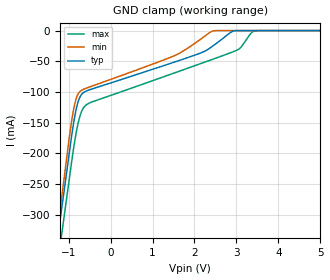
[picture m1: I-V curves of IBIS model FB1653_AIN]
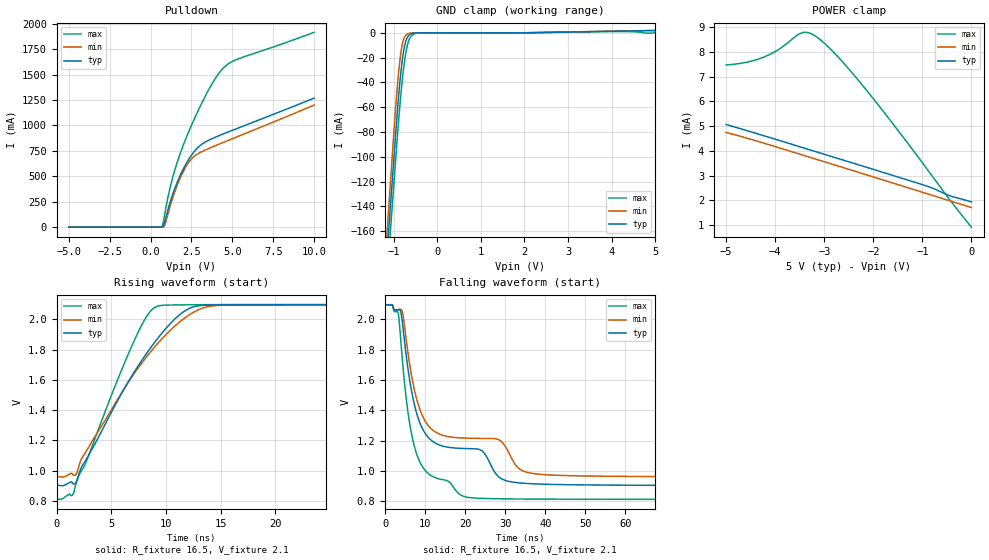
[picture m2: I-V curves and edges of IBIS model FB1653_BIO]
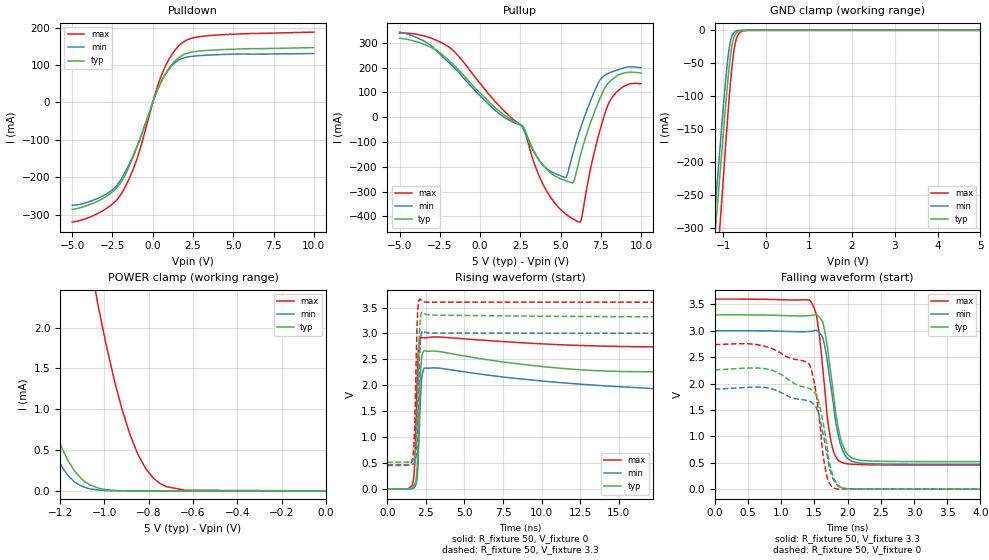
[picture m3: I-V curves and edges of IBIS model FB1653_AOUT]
| TEXAS INSTRUMENTS INCORPORATED
| Standard Linear and Logic Group
| IBIS Model of SN74FB1653
| 17-BIT LVTTL/BTL UNIVERSAL STORAGE TRANSCEIVER WITH BUFFERED CLOCK
| LINE
| This file contains package information for the following:
|  TQFP 100-pin (PCA) package as [Component] FB1653_PCA
| This device can be powered at the following Vccs:
|  5 volt Vcc
| This file provides unique models under the [Model Selector] for each Vcc.
| For operation at a specific Vcc, select the appropriate model after each
| [Model Selector] keyword.
[IBIS Ver]   3.2
[Comment char]  |_char
[File Name]   sn74fb1653.ibs
[File Rev]   1.1 | x_die
[Date]   December 15, 2005
[Source]   Data created from TI-SPICE simulations at TI-SLL.
[Notes]   The following is an IBIS list for the FB1653.
   Please contact sllibis@ti.com with questions and
   comments concerning SLL IBIS models.
   This IBIS model is created from a BA (back annotated netlist)
   - FILE REV HISTORY
   - 1.1 Release IBIS file on 12/19/05
   - Non-monotonic data in output due to feedback circuit
   - Non-monotonic data in pullup data due to damping resistor.
   - End point warning due to AC and DC mismatch.
   - Power Clamp never becomes zero due to internal
   pulldown resistors.
   - Power clamp data deleted in AIN model as there is no
   power-clamp diode.
   - Process for this device is BiCMOS which relates to some of
   the unusual curves and reversal of temperatures vs min/max
   values vs a CMOS device.
[Disclaimer] Property of Texas Instruments Incorporated.  Unauthorized
   reproduction and/or distribution is strictly prohibited.
   This product is protected under copyright law.
   Created  2005, (C) Copyright  2005, Texas Instruments
   Incorporated, All Rights Reserved
   UNLESS THERE IS A SIGNED, WRITTEN AGREEMENT TO THE
   CONTRARY, TEXAS INSTRUMENTS (TI) IS PROVIDING THE IBIS
   MODELS  AND WITHOUT ANY WARRANTY, EXPRESSED OR
   IMPLIED.  TI assumes no liability for:
   1) the accuracy of the IBIS models provided to your
   company;
   2) the proper functioning of these IBIS Models in your
   design or for any resulting applications; or
   3) infringement of patents, copyrights or intellectual
   property rights resulting from your use of these IBIS
   models.
   TI provides IBIS Models as a service to our customers.
   You and your company shall not distribute, sell or give
   these models to anyone else without prior written
   permission from TI.
   TI reserves the right to make changes to our products or
   to discontinue any semiconductor product or service
   without notice, and advises our customers to obtain the
   latest version of relevant information to verify, before
   placing orders, that the information being relied on is
   current.
   Please be aware that your receipt and use of the IBIS
   information provided shall serve as acceptance of these
   terms and conditions.  If you do not accept these terms,
   you should return or destroy the IBIS models and any
   other accompanying information immediately.
| Component FB1653_PCA 100-pin TQFP
[Component]   FB1653_PCA
[Manufacturer]   Texas Instruments, Inc.
[Package]
|   typ   min   max
R_pkg   7.100e-02   6.300e-02   7.700e-02
L_pkg   4.124e-09   3.790e-09   4.624e-09
C_pkg   4.380e-13   3.540e-13   6.860e-13
[Pin]   signal_name   model_name   R_pin   L_pin   C_pin
1   VCC33   POWER   6.500e-02   4.623e-09   6.860e-13
2   VCC   POWER   6.300e-02   4.403e-09   5.280e-13
3   GND   GND   6.700e-02   4.343e-09   4.930e-13
4   1AO6   FB1653_AOUT   6.700e-02   4.242e-09   4.650e-13
5   1AI6   FB1653_AIN   7.000e-02   4.182e-09   4.420e-13
6   1AO7   FB1653_AOUT   7.100e-02   4.118e-09   4.220e-13
7   1AI7   FB1653_AIN   7.200e-02   4.067e-09   4.110e-13
8   GND   GND   7.300e-02   3.998e-09   3.930e-13
9   1AO8   FB1653_AOUT   7.400e-02   3.962e-09   3.720e-13
10   1AI8   FB1653_AIN   7.500e-02   3.932e-09   3.650e-13
11   1AO9   FB1653_AOUT   7.500e-02   3.902e-09   3.560e-13
12   1AI9   FB1653_AIN   7.700e-02   3.888e-09   3.540e-13
13   GND   GND   7.600e-02   3.790e-09   3.670e-13
14   2CLK   FB1653_AOUT   7.600e-02   3.887e-09   3.590e-13
15   VCC33   POWER   7.500e-02   3.901e-09   3.560e-13
16   2AO2   FB1653_AOUT   7.500e-02   3.933e-09   3.650e-13
17   2AI2   FB1653_AIN   7.500e-02   3.962e-09   3.720e-13
18   GND   GND   7.300e-02   3.999e-09   3.930e-13
19   2AO3   FB1653_AOUT   7.300e-02   4.068e-09   4.110e-13
20   2AI3   FB1653_AIN   7.100e-02   4.119e-09   4.220e-13
21   2AO4   FB1653_AOUT   7.000e-02   4.182e-09   4.420e-13
22   2AI4   FB1653_AIN   6.600e-02   4.241e-09   4.650e-13
23   GND   GND   6.700e-02   4.342e-09   4.930e-13
24   VCC   POWER   6.300e-02   4.402e-09   5.280e-13
25   VCC33   POWER   6.600e-02   4.623e-09   6.860e-13
26   2AO5   FB1653_AOUT   6.500e-02   4.623e-09   6.850e-13
27   2AI5   FB1653_AIN   6.300e-02   4.402e-09   5.280e-13
28   2AO6   FB1653_AOUT   6.700e-02   4.343e-09   4.930e-13
29   2AI6   FB1653_AIN   6.600e-02   4.241e-09   4.650e-13
30   GND   GND   6.900e-02   4.181e-09   4.420e-13
31   2AO7   FB1653_AOUT   7.000e-02   4.118e-09   4.220e-13
32   2AI7   FB1653_AIN   7.200e-02   4.067e-09   4.110e-13
33   2AO8   FB1653_AOUT   7.300e-02   3.998e-09   3.930e-13
34   2AI8   FB1653_AIN   7.400e-02   3.962e-09   3.720e-13
35   GND   GND   7.500e-02   3.932e-09   3.650e-13
36   2AO9   NC   7.500e-02   3.902e-09   3.560e-13
37   2AI9   FB1653_AIN   7.500e-02   3.885e-09   3.550e-13
38   VCC   POWER   7.600e-02   3.790e-09   3.670e-13
39   2OEA   NC   7.500e-02   3.885e-09   3.600e-13
40   2OEA_BAR   NC   7.500e-02   3.901e-09   3.560e-13
41   2LEBA   NC   7.500e-02   3.932e-09   3.650e-13
42   2CLKBA   NC   7.500e-02   3.962e-09   3.720e-13
43   2CLKAB   NC   7.200e-02   3.997e-09   3.930e-13
44   2LEAB   NC   7.300e-02   4.068e-09   4.110e-13
45   2OEB   NC   7.100e-02   4.118e-09   4.220e-13
46   2OEB_BAR   NC   7.000e-02   4.182e-09   4.420e-13
47   BIAS_VCC   NC   6.700e-02   4.243e-09   4.650e-13
48   2SEL1   NC   6.700e-02   4.342e-09   4.930e-13
49   GND   GND   6.300e-02   4.402e-09   5.280e-13
50   2B9_BAR   FB1653_BIO   6.600e-02   4.623e-09   6.860e-13
51   2B8_BAR   FB1653_BIO   6.500e-02   4.623e-09   6.850e-13
52   GND   GND   6.300e-02   4.403e-09   5.280e-13
53   2B7_BAR   FB1653_BIO   6.700e-02   4.343e-09   4.930e-13
54   2B6_BAR   FB1653_BIO   6.700e-02   4.241e-09   4.650e-13
55   GND   GND   7.000e-02   4.182e-09   4.420e-13
56   2B5_BAR   FB1653_BIO   7.100e-02   4.118e-09   4.220e-13
57   2B4_BAR   FB1653_BIO   7.200e-02   4.067e-09   4.110e-13
58   GND   GND   7.300e-02   3.998e-09   3.930e-13
59   2B3_BAR   FB1653_BIO   7.400e-02   3.962e-09   3.720e-13
60   2B2_BAR   FB1653_BIO   7.500e-02   3.932e-09   3.650e-13
61   GND   GND   7.500e-02   3.902e-09   3.560e-13
62   2CLKAB_BAR NC   7.700e-02   3.888e-09   3.540e-13
63   2SEL2   NC   7.600e-02   3.790e-09   3.670e-13
64   1B9_BAR   FB1653_BIO   7.600e-02   3.887e-09   3.590e-13
65   GND   GND   7.500e-02   3.901e-09   3.560e-13
66   1B8_BAR   FB1653_BIO   7.500e-02   3.932e-09   3.650e-13
67   1B7_BAR   FB1653_BIO   7.500e-02   3.962e-09   3.720e-13
68   GND   GND   7.300e-02   3.999e-09   3.930e-13
69   1B6_BAR   FB1653_BIO   7.300e-02   4.068e-09   4.110e-13
70   1B5_BAR   FB1653_BIO   7.100e-02   4.119e-09   4.220e-13
71   GND   GND   7.000e-02   4.182e-09   4.420e-13
72   1B4_BAR   FB1653_BIO   6.600e-02   4.241e-09   4.650e-13
73   1B3_BAR   FB1653_BIO   6.700e-02   4.342e-09   4.930e-13
74   GND   GND   6.300e-02   4.402e-09   5.280e-13
75   1B2_BAR   FB1653_BIO   6.600e-02   4.624e-09   6.860e-13
76   1B1_BAR   FB1653_BIO   6.500e-02   4.623e-09   6.850e-13
77   BG_GND   GND   6.300e-02   4.402e-09   5.280e-13
78   BG_VCC   NC   6.700e-02   4.343e-09   4.930e-13
79   VREF   NC   6.700e-02   4.242e-09   4.650e-13
80   1OEB_BAR   NC   6.900e-02   4.181e-09   4.420e-13
81   1OEB   NC   7.100e-02   4.119e-09   4.220e-13
82   1LEAB   NC   7.200e-02   4.067e-09   4.110e-13
83   1CLKAB   NC   7.300e-02   3.998e-09   3.930e-13
84   1CLKBA   NC   7.400e-02   3.962e-09   3.720e-13
85   1LEBA   NC   7.500e-02   3.932e-09   3.650e-13
86   1OEA_BAR   NC   7.500e-02   3.902e-09   3.560e-13
87   1OEA   NC   7.500e-02   3.885e-09   3.550e-13
88   VCC   POWER   7.600e-02   3.790e-09   3.670e-13
89   1AO1   FB1653_AOUT   7.500e-02   3.885e-09   3.600e-13
90   1AI1   FB1653_AIN   7.500e-02   3.901e-09   3.560e-13
91   GND   GND   7.400e-02   3.930e-09   3.650e-13
92   1AO2   FB1653_AOUT   7.500e-02   3.962e-09   3.720e-13
93   1AI2   FB1653_AIN   7.200e-02   3.997e-09   3.930e-13
94   1AO3   FB1653_AOUT   7.300e-02   4.068e-09   4.110e-13
95   1AI3   FB1653_AIN   7.100e-02   4.118e-09   4.220e-13
96   GND   GND   7.000e-02   4.182e-09   4.420e-13
97   1AO4   FB1653_AOUT   6.700e-02   4.243e-09   4.650e-13
98   1AI4   FB1653_AIN   6.700e-02   4.342e-09   4.930e-13
99   1AO5   FB1653_AOUT   6.300e-02   4.402e-09   5.280e-13
100   1AI5   FB1653_AIN   6.600e-02   4.624e-09   6.860e-13
| Models and submodels in the file (3): FB1653_AIN (Input), FB1653_BIO (I/O_open_drain), FB1653_AOUT (3-state)
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[Model]   FB1653_AIN
Model_type  Input
Vinl=0.8
Vinh=2.0
| variable   typ   min   max
C_comp   3.25pF   2.53pF   4.61pF
[Temperature Range]   40   0   85
| Ambient temperature   25   0   70
[Voltage range]   5   4.5   5.5
[GND Clamp]
| FB1653_AIN
|   Voltage   I(typ)   I(min)   I(max)
-5V       -2.211A    -2.34A     -2.239A
-1.51V    -464mA     -459.1mA   -504.4mA
-1V       -208.1mA   -183.3mA   -250.3mA
-850mV    -139mA     -118.9mA   -179.1mA
-775mV    -116.6mA   -103.6mA   -151.8mA
-700mV    -104.8mA   -97.7mA    -133.4mA
-475mV    -95.8mA    -91.21mA   -117.1mA
1.55V     -50.61mA   -40.03mA   -68.29mA
2.44V     -24.94mA   -668.5uA   -46.55mA
3.065V    -7.924uA   1.877pA    -29.76mA
3.43V     -5.268pA   2.985pA    -630.6uA
5V        17.18pA    8.04pA     105.7pA
[Model]   FB1653_BIO
Model_type  I/O_open_drain
Vinl=1.47
Vinh=1.62
Enable   Active-Low
Vref =   2.1
Rref =   16.5
Cref =   30p
Vmeas =   1.55
| variable   typ   min   max
C_comp   7.67pF   5.68pF   11.34pF
| C_pulldown   136.63pF   3.54pF   271.38pF
| C_tri-state   7.67pF   5.68pF   11.34pF
[Temperature Range]   40   0   85
| Ambient temperature   25   0   70
[Voltage range]   5   4.5   5.5
[Pullup Reference]   5   5   5
[POWER Clamp Reference]   5   5   5
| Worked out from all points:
|   slope of the pulldown table from 0 to 0.75 V, typ, clamps not added: 163 ohm
|   GND clamp passes 1 mA (typ) near -0.62 V on its own axis
|   rising waveform, R_fixture 16.5, V_fixture 2.1: 20-80 % time 5.84ns typ, 6.41ns min, 4.21ns max; typ from 0.903 V to 2.1 V
|   falling waveform, R_fixture 16.5, V_fixture 2.1: 20-80 % time 18.5ns typ, 24ns min, 4.53ns max; typ from 2.1 V to 0.903 V
[GND Clamp]
| FB1653_BIO
|   Voltage   I(typ)   I(min)   I(max)
-5V       -2.029A    -2.154A    -2.028A
-1.195V   -195.3mA   -180.9mA   -214.8mA
-1.145V   -171.2mA   -155mA     -190.9mA
-1.09V    -144.7mA   -126.5mA   -164.7mA
-975mV    -89.23mA   -67.4mA    -109.9mA
-875mV    -44.36mA   -26.02mA   -63.76mA
-825mV    -26.99mA   -12.68mA   -44.23mA
-775mV    -14.36mA   -5.177mA   -28.17mA
-675mV    -2.644mA   -568.7uA   -7.913mA
-575mV    -332.9uA   -24.17uA   -1.561mA
-425mV    -3.755uA   -351.3nA   -70.94uA
5V        1.944mA    2.018mA    20.13uA
[POWER Clamp]
| FB1653_BIO
|   Voltage   I(typ)   I(min)   I(max)
-5V       5.068mA    4.747mA    7.476mA
-4.57V    4.818mA    4.514mA    7.593mA
-4.195V   4.593mA    4.293mA    7.825mA
-3.93V    4.433mA    4.133mA    8.103mA
-3.455V   4.144mA    3.843mA    8.775mA
-3.33V    4.067mA    3.767mA    8.783mA
-3.18V    3.976mA    3.675mA    8.643mA
-2.785V   3.734mA    3.432mA    7.94mA
-2.195V   3.373mA    3.068mA    6.591mA
-920mV    2.586mA    2.281mA    3.306mA
-445mV    2.19mA     1.984mA    2.034mA
-84.45fV  1.939mA    1.711mA    918.5uA
[Pulldown]
| FB1653_BIO
|   Voltage   I(typ)   I(min)   I(max)
-5V       266uA      831uA      515uA
670mV     382.3uA    120.9uA    4.223mA
755mV     5.331mA    575uA      34.2mA
870mV     52.71mA    20.99mA    131mA
1.12V     203.8mA    164mA      337.2mA
1.415V    351.5mA    318.1mA    524.5mA
1.865V    527.2mA    502.1mA    748.2mA
2.315V    661.7mA    633.2mA    932.6mA
3.065V    806.6mA    736.4mA    1.198A
4.22V     901.7mA    818.2mA    1.521A
5.175V    962.9mA    880.7mA    1.642A
10V       1.268A     1.2A       1.915A
[Ramp]
| FB1653_BIO
| variable   typ   min   max
dV/dt_r   0.72/5.85E-09   0.68/6.42E-09   0.77/4.22E-09
dV/dt_f   0.72/1.86E-08   0.68/2.40E-08   0.77/4.52E-09
R_load = 16.5
[Rising Waveform]
| FB1653_BIO
R_fixture =   16.5
C_fixture =   0
L_fixture =   0
V_fixture =   2.1
V_fixture_min = 2.1
V_fixture_max = 2.1
|   Time   V(typ)   V(min)   V(max)
0s        902.6mV    960mV      811.6mV
1.525ns   912.2mV    971.7mV    846.2mV
1.915ns   942.5mV    998.8mV    948.6mV
2.365ns   1.034V     1.088V     1.009V
7.14ns    1.656V     1.646V     1.866V
8.425ns   1.795V     1.77V      2.039V
9.415ns   1.89V      1.854V     2.091V
12.03ns   2.068V     2.025V     2.097V
14.99ns   2.095V     2.093V     2.098V
95ns      2.097V     2.096V     2.099V
[Falling Waveform]
| FB1653_BIO
R_fixture =   16.5
C_fixture =   0
L_fixture =   0
V_fixture =   2.1
V_fixture_min = 2.1
V_fixture_max = 2.1
|   Time   V(typ)   V(min)   V(max)
0s        2.097V     2.096V     2.099V
3.24ns    2.063V     2.065V     2.041V
4.32ns    1.975V     2.048V     1.725V
5.665ns   1.678V     1.784V     1.391V
8.24ns    1.347V     1.439V     1.084V
11.96ns   1.192V     1.267V     961.2mV
19.05ns   1.148V     1.217V     837.4mV
28.38ns   960mV      1.205V     815.2mV
32.53ns   922.9mV    1.04V      814mV
95ns      903.2mV    960.7mV    811.6mV
[Model]   FB1653_AOUT
Model_type  3-state
Enable   Active-Low
Vref =   0
Rref =   500
Cref =   50p
Vmeas =   1.5
| variable   typ   min   max
C_comp   3.31pF   2.65pF   4.60pF
| C_pullup   14.00pF   2.17pF   31.38pF
| C_pulldown   4.54pF   3.52pF   5.52pF
| C_tri-state   3.31pF   2.65pF   4.60pF
[Temperature Range]   40   0   85
| Ambient temperature   25   0   70
[Voltage range]   5   4.5   5.5
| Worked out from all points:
|   slope of the pulldown table from 0 to 0.75 V, typ, clamps not added: 10.1 ohm
|   slope of the pullup table from 0 to 0.75 V, typ, clamps not added: 15.6 ohm
|   GND clamp passes 1 mA (typ) near -0.62 V on its own axis
|   POWER clamp passes 1 mA (typ) near -1.25 V on its own axis
|   rising waveform, R_fixture 50, V_fixture 0: 20-80 % time 150ps typ, 142ps min, 158ps max; typ from 0 V to 2.26 V
|   falling waveform, R_fixture 50, V_fixture 3.3: 20-80 % time 184ps typ, 181ps min, 156ps max; typ from 3.3 V to 0.521 V
|   rising waveform, R_fixture 50, V_fixture 3.3: 20-80 % time 149ps typ, 146ps min, 153ps max; typ from 0.52 V to 3.3 V
|   falling waveform, R_fixture 50, V_fixture 0: 20-80 % time 217ps typ, 194ps min, 175ps max; typ from 2.26 V to 0 V
[GND Clamp]
| FB1653_AOUT
|   Voltage   I(typ)   I(min)   I(max)
-5V       -2.918A    -3.081A    -3.124A
-1.245V   -349.6mA   -314.7mA   -445.1mA
-1.21V    -322.6mA   -286.5mA   -414.7mA
-1.18V    -299.4mA   -262.3mA   -388.3mA
-1.065V   -209.2mA   -169.4mA   -285.5mA
-975mV    -138.1mA   -97.9mA    -203.2mA
-890mV    -74.3mA    -41.42mA   -126.4mA
-800mV    -24.76mA   -8.897mA   -57.28mA
-700mV    -4.377mA   -1.072mA   -14.24mA
-625mV    -1.02mA    -142.5uA   -4.11mA
-450mV    -9.008uA   -781.8nA   -161.9uA
5V        76.3nA     81.14nA    192.5nA
[POWER Clamp]
| FB1653_AOUT
|   Voltage   I(typ)   I(min)   I(max)
-5V       157.4mA    171.9mA    187.5mA
-1.41V    2.872mA    2.535mA    9.974mA
-1.38V    2.444mA    2.091mA    9.219mA
-1.32V    1.681mA    1.324mA    7.777mA
-1.24V    877.2uA    577.6uA    6.006mA
-1.165V   373.8uA    189.5uA    4.514mA
-1.07V    79.76uA    28.17uA    2.883mA
-1.03V    36.02uA    11.13uA    2.291mA
-885mV    1.121uA    199.7nA    693.7uA
-780mV    55.56nA    7.616nA    158.2uA
-635mV    1.15nA     226.3pA    8.446uA
-84.45fV  325.1pA    116pA      45.91nA
[Pulldown]
| FB1653_AOUT
|   Voltage   I(typ)   I(min)   I(max)
-5V       -286.3mA   -275.3mA   -320.3mA
-2.975V   -254mA     -247.2mA   -286.1mA
-2.345V   -233mA     -227.7mA   -265.6mA
-1.915V   -209.9mA   -201.8mA   -241.8mA
-1.425V   -167mA     -161.3mA   -200.2mA
-965mV    -118.7mA   -116.4mA   -149.2mA
140mV     17.02mA    17mA       21.69mA
560mV     59.06mA    58.32mA    74.7mA
1.155V    99.85mA    96.71mA    125.9mA
1.815V    125.4mA    117.5mA    159mA
3.565V    139.7mA    126.8mA    178.9mA
10V       146.6mA    130.6mA    188.2mA
[Pullup]
| FB1653_AOUT
|   Voltage   I(typ)   I(min)   I(max)
-5V       319mA      343.3mA    339.7mA
-1.57V    206.3mA    197.8mA    263.1mA
2.67V     -37.61mA   -45.73mA   -42.42mA
3.545V    -159mA     -162.3mA   -217.6mA
4.39V     -225.4mA   -218.5mA   -323.9mA
5.35V     -257.3mA   -241.7mA   -392.2mA
5.8V      -262.9mA   -138.6mA   -411.3mA
6.16V     -173.1mA   -59.95mA   -423.7mA
7.315V    55.42mA    134.5mA    -84.24mA
7.96V     136.8mA    177mA      51.65mA
8.88V     177.4mA    197.7mA    122.4mA
10V       178.1mA    199.2mA    134.8mA
[Ramp]
| FB1653_AOUT
| variable   typ   min   max
dV/dt_r   1.60/1.86E-10   1.40/1.83E-10   1.76/1.76E-10
dV/dt_f   1.67/1.94E-10   1.52/1.93E-10   1.89/1.71E-10
R_load = 50
[Rising Waveform]
| FB1653_AOUT
R_fixture =   50
C_fixture =   0
L_fixture =   0
V_fixture =   0
V_fixture_min = 0
V_fixture_max = 0
|   Time   V(typ)   V(min)   V(max)
0s        959.2pV    789.6pV    4.036nV
1.645ns   37.66mV    10.52mV    116.1mV
1.78ns    101.3mV    48.55mV    545.3mV
1.915ns   369.8mV    178.3mV    1.973V
2.025ns   1.235V     773.4mV    2.734V
2.185ns   2.419V     1.962V     2.922V
2.37ns    2.667V     2.322V     2.915V
3.015ns   2.661V     2.337V     2.933V
21.01ns   2.259V     1.905V     2.737V
95ns      2.259V     1.893V     2.736V
[Falling Waveform]
| FB1653_AOUT
R_fixture =   50
C_fixture =   0
L_fixture =   0
V_fixture =   3.3
V_fixture_min = 3.0
V_fixture_max = 3.6
|   Time   V(typ)   V(min)   V(max)
0s        3.3V       3V         3.6V
1.43ns    3.287V     2.987V     3.58V
1.53ns    3.305V     3.008V     3.299V
1.625ns   3.167V     2.876V     2.31V
1.705ns   2.606V     2.336V     1.269V
1.79ns    1.779V     1.574V     709.4mV
1.87ns    1.098V     965.3mV    535.8mV
1.955ns   747.9mV    661.4mV    491mV
2.255ns   539.8mV    487.8mV    463.3mV
95ns      521.5mV    471.2mV    456.1mV
[Rising Waveform]
| FB1653_AOUT
R_fixture =   50
C_fixture =   0
L_fixture =   0
V_fixture =   3.3
V_fixture_min = 3.0
V_fixture_max = 3.6
|   Time   V(typ)   V(min)   V(max)
0s        520.2mV    470.2mV    454.5mV
1.625ns   536.8mV    478.9mV    576.3mV
1.75ns    609.2mV    508.2mV    1.068V
1.875ns   916.3mV    697mV      2.618V
1.97ns    1.849V     1.292V     3.445V
2.055ns   2.825V     2.261V     3.638V
2.11ns    3.177V     2.699V     3.663V
2.19ns    3.378V     2.977V     3.643V
2.315ns   3.407V     3.047V     3.614V
95ns      3.302V     3.001V     3.6V
[Falling Waveform]
| FB1653_AOUT
R_fixture =   50
C_fixture =   0
L_fixture =   0
V_fixture =   0
V_fixture_min = 0
V_fixture_max = 0
|   Time   V(typ)   V(min)   V(max)
0s        2.262V     1.896V     2.739V
795ps     2.274V     1.919V     2.692V
1.425ns   1.905V     1.669V     2.368V
1.49ns    1.847V     1.606V     2.071V
1.55ns    1.718V     1.473V     1.593V
1.625ns   1.308V     1.08V      702.7mV
1.685ns   862.9mV    696.6mV    261.4mV
1.76ns    340.3mV    264mV      50.32mV
1.865ns   70.09mV    53.35mV    1.2mV
95ns      731.3nV    606.2nV    760.8nV
